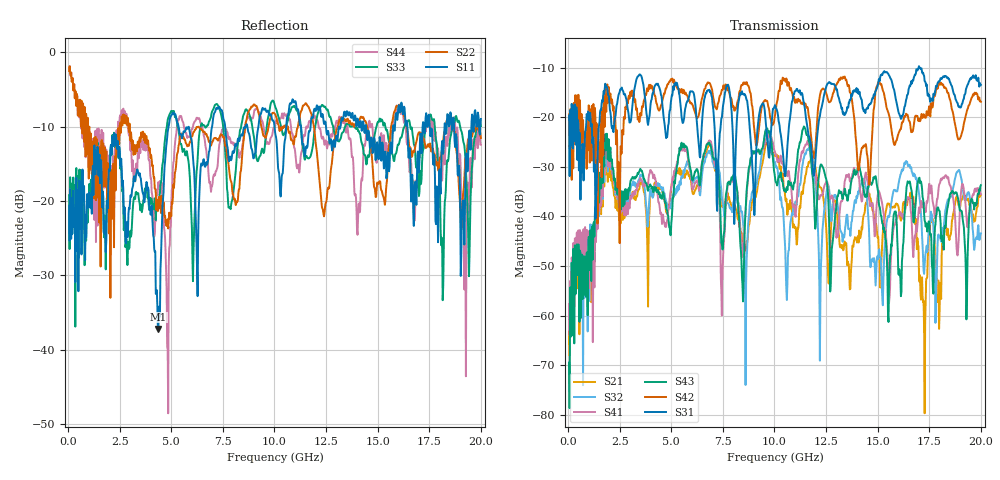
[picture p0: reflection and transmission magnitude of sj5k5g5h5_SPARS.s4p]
! FILE: E:\users\goganessyan\GBX_Backplane\FR408_backplane\1m_INBOUND_NEXT\sj5k5g5h5_SPARS.s4p
# MHZ S RI R 50.00
! FREQ  S11  S12  S13  S14
!  S21  S22  S23  S24
!  S31  S32  S33  S34
!  S41  S42  S43  S44
!  REAL  IMAG  REAL  IMAG  REAL  IMAG  REAL  IMAG
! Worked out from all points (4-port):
!   799 points, 50 MHz to 20 GHz, reference 50 ohm
!   strongest paths, dB at 50 MHz, 5.025 GHz, 10.03 GHz, 15.03 GHz, 20 GHz:
!     S31: -19.6, -15.6, -17.5, -13.2, -13.4
!     S42: -19.4, -12.5, -19.6, -12.9, -16.8
!     S43: -69.5, -40.2, -32.1, -35.2, -33.7
!     S41: -57.7, -33.8, -27.0, -35.0, -35.5
!     S32: -60.8, -36.6, -29.0, -48.6, -43.4
!     S21: -63.2, -33.3, -27.8, -44.1, -35.6
!   lowest |S11| = -37.2 dB at 4.375 GHz (marker M1), VSWR 1.03, Z = 50.1 + j1.38 ohm
!   |S11| at or under -10 dB: start of sweep to 4.875 GHz; 5.35 GHz to 6.978 GHz (1.628 GHz wide, 26.4 % of centre); 14.43 GHz to 15.75 GHz (1.314 GHz wide, 8.71 % of centre)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
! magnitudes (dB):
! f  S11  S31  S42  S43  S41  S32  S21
! 50 MHz  -20.7  -19.6  -19.4  -69.5  -57.7  -60.8  -63.2
! 1.8 GHz  -23.9  -13.2  -14.9  -23.4  -24.4  -25.3  -26.3
! 4.375 GHz  -37.2  -13.5  -18.4  -35.3  -37.1  -33.9  -34.7
! 5.05 GHz  -8.3  -15.6  -12.2  -38.5  -32.7  -36.6  -32.9
! 16.65 GHz  -17.2  -13.2  -23.0  -35.0  -41.3  -31.0  -36.0
! 17.25 GHz  -10.7  -11.6  -19.8  -39.5  -38.2  -51.6  -63.3
! 20 GHz  -9.0  -13.4  -16.8  -33.7  -35.5  -43.4  -35.6
